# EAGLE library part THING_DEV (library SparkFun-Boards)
SparkFun Thing -Dev Board The SparkFun ESP8266 Thing Dev is a breakout and development board for the ESP8266 WiFi SoC, with an integrated FTDI USB-to-Serial chip. SparkFun Products: SparkFun ESP8266 Thing-Dev Board
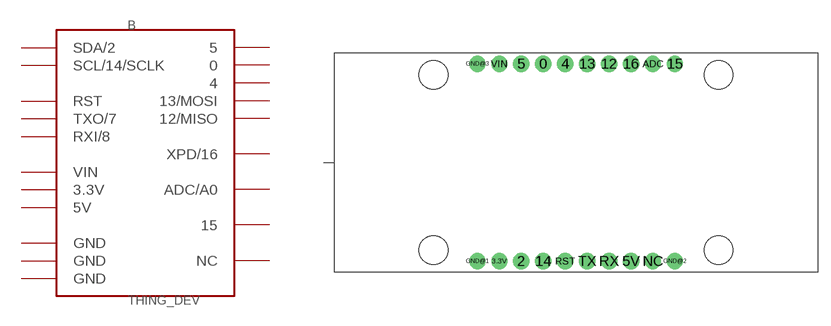
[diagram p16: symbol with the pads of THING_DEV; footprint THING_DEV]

Designator prefix B

## THING_DEV (SF_ID: WRL-13711)  [THING_DEV]
0  0
2  SDA/2
3.3V  3.3V  pwr
4  4
5  5
5V  5V  pwr
12  12/MISO
13  13/MOSI
14  SCL/14/SCLK
15  15
16  XPD/16
ADC  ADC/A0
GND@1  GND  pwr
GND@2  GND  pwr
GND@3  GND  pwr
NC  NC  nc
RST  RST  in
RX  RXI/8  in
TX  TXO/7  out
VIN  VIN  pwr

## Footprint THING_DEV (pad centres in mm)
SparkFun Thing Board Footprint Specifications: Pin count: 20 Pin pitch:0.1 inch Area: 2.2 x 1.0 inchees
drill 1.016 pad 1.88: 0 24.13,24.13; 2 21.59,1.27; 3.3V 19.05,1.27; 4 26.67,24.13; 5 21.59,24.13; 5V 34.29,1.27; 12 31.75,24.13; 13 29.21,24.13; 14 24.13,1.27; 15 39.37,24.13; 16 34.29,24.13; ADC 36.83,24.13; GND@1 16.51,1.27; GND@2 39.37,1.27; GND@3 16.51,24.13; NC 36.83,1.27; RST 26.67,1.27; RX 31.75,1.27; TX 29.21,1.27; VIN 19.05,24.13
hole 3.302 at 11.43,2.54
hole 3.302 at 11.43,22.86
hole 3.302 at 44.45,22.86
hole 3.302 at 44.45,2.54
